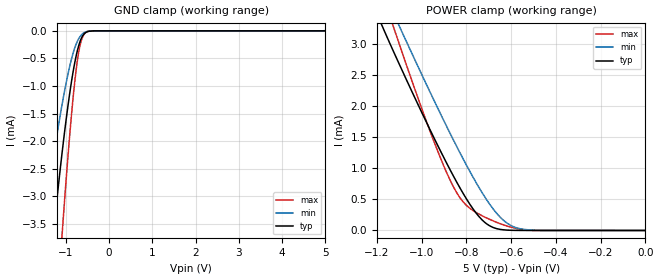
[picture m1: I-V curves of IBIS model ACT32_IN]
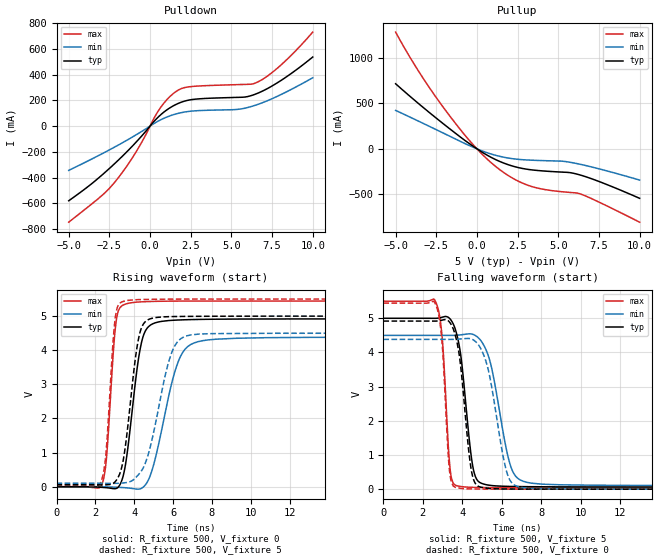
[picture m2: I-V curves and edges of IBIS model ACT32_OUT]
| TEXAS INSTRUMENTS INCORPORATED
| Standard Linear and Logic Group
| IBIS Model of SN74ACT32
| QUADRUPLE 2-INPUT POSITIVE-OR GATES
| This file contains package information for the following:
|  SOIC 14-pin (D) package as [Component] ACT32_D
|  SSOP 14-pin (DB) package as [Component] ACT32_DB
|  PDIP 14-pin (N) package as [Component] ACT32_N
|  TSSOP 14-pin (PW) package as [Component] ACT32_PW
| This device can be powered at the following Vccs:
|  5 volt Vcc
| This file provides unique models under the [Model Selector] for each Vcc.
| For operation at a specific Vcc, select the appropriate model after each
| [Model Selector] keyword.
[IBIS Ver]   3.2
[Comment char]  |_char
[File Name]   sn74act32.ibs
[File Rev]   1.1 | x_die
[Date]   September 5, 2002
[Source]   Data created from TI-SPICE simulations at TI-SLL.
[Notes]   The following is an IBIS list for the ACT32.
   Please contact sllibis@ti.com with questions and
   comments concerning SLL IBIS models.
   This IBIS model is created from a BA (back annotated netlist
[Disclaimer] Property of Texas Instruments Incorporated.  Unauthorized
   reproduction and/or distribution is strictly prohibited.
   This product is protected under copyright law.
   Created  2002, (C) Copyright  2002, Texas Instruments
   Incorporated, All Rights Reserved
   UNLESS THERE IS A SIGNED, WRITTEN AGREEMENT TO THE
   CONTRARY, TEXAS INSTRUMENTS (TI) IS PROVIDING THE IBIS
   MODELS  AND WITHOUT ANY WARRANTY, EXPRESSED OR
   IMPLIED.  TI assumes no liability for:
   1) the accuracy of the IBIS models provided to your
   company;
   2) the proper functioning of these IBIS Models in your
   design or for any resulting applications; or
   3) infringement of patents, copyrights or intellectual
   property rights resulting from your use of these IBIS
   models.
   TI provides IBIS Models as a service to our customers.
   You and your company shall not distribute, sell or give
   these models to anyone else without prior written
   permission from TI.
   TI reserves the right to make changes to our products or
   to discontinue any semiconductor product or service
   without notice, and advises our customers to obtain the
   latest version of relevant information to verify, before
   placing orders, that the information being relied on is
   current.
   Please be aware that your receipt and use of the IBIS
   information provided shall serve as acceptance of these
   terms and conditions.  If you do not accept these terms,
   you should return or destroy the IBIS models and any
   other accompanying information immediately.
| Component ACT32_D 14-pin SOIC
[Component]   ACT32_D
[Manufacturer]   Texas Instruments, Inc.
[Package]
|   typ   min   max
R_pkg   3.100e-02   2.800e-02   3.400e-02
L_pkg   3.109e-09   2.462e-09   3.889e-09
C_pkg   4.730e-13   3.630e-13   6.280e-13
[Pin]   signal_name   model_name   R_pin   L_pin   C_pin
1   1A   ACT32_IN   3.300e-02   3.854e-09   6.220e-13
2   1B   ACT32_IN   3.200e-02   3.188e-09   4.730e-13
3   1Y   ACT32_OUT   2.800e-02   2.462e-09   3.770e-13
4   2A   ACT32_IN   3.100e-02   2.596e-09   3.630e-13
5   2B   ACT32_IN   2.800e-02   2.521e-09   3.720e-13
6   2Y   ACT32_OUT   3.400e-02   3.250e-09   4.760e-13
7   GND   GND   3.400e-02   3.889e-09   6.280e-13
8   3Y   ACT32_OUT   3.400e-02   3.889e-09   6.280e-13
9   3A   ACT32_IN   3.400e-02   3.250e-09   4.760e-13
10   3B   ACT32_IN   2.800e-02   2.521e-09   3.720e-13
11   4Y   ACT32_OUT   3.100e-02   2.596e-09   3.640e-13
12   4A   ACT32_IN   2.800e-02   2.462e-09   3.770e-13
13   4B   ACT32_IN   3.200e-02   3.188e-09   4.730e-13
14   VCC   POWER   3.300e-02   3.854e-09   6.220e-13
| Component ACT32_DB 14-pin SSOP
[Component]   ACT32_DB
[Manufacturer]   Texas Instruments, Inc.
[Package]
|   typ   min   max
R_pkg   4.400e-02   4.100e-02   4.600e-02
L_pkg   3.551e-09   3.258e-09   3.927e-09
C_pkg   4.020e-13   3.600e-13   4.210e-13
[Pin]   signal_name   model_name   R_pin   L_pin   C_pin
1   1A   ACT32_IN   4.600e-02   3.927e-09   4.080e-13
2   1B   ACT32_IN   4.400e-02   3.587e-09   4.210e-13
3   1Y   ACT32_OUT   4.100e-02   3.289e-09   3.980e-13
4   2A   ACT32_IN   4.200e-02   3.258e-09   3.600e-13
5   2B   ACT32_IN   4.100e-02   3.286e-09   4.030e-13
6   2Y   ACT32_OUT   4.400e-02   3.586e-09   4.210e-13
7   GND   GND   4.600e-02   3.927e-09   4.080e-13
8   3Y   ACT32_OUT   4.600e-02   3.927e-09   4.080e-13
9   3A   ACT32_IN   4.400e-02   3.586e-09   4.210e-13
10   3B   ACT32_IN   4.100e-02   3.286e-09   4.030e-13
11   4Y   ACT32_OUT   4.300e-02   3.258e-09   3.600e-13
12   4A   ACT32_IN   4.100e-02   3.289e-09   3.980e-13
13   4B   ACT32_IN   4.400e-02   3.587e-09   4.210e-13
14   VCC   POWER   4.600e-02   3.927e-09   4.080e-13
| Component ACT32_N 14-pin PDIP
[Component]   ACT32_N
[Manufacturer]   Texas Instruments, Inc.
[Package]
|   typ   min   max
R_pkg   4.500e-02   3.700e-02   6.300e-02
L_pkg   5.407e-09   3.922e-09   6.942e-09
C_pkg   3.890e-13   2.050e-13   6.040e-13
[Pin]   signal_name   model_name   R_pin   L_pin   C_pin
1   1A   ACT32_IN   6.300e-02   6.942e-09   6.040e-13
2   1B   ACT32_IN   3.700e-02   6.200e-09   4.060e-13
3   1Y   ACT32_OUT   4.200e-02   4.389e-09   3.220e-13
4   2A   ACT32_IN   3.800e-02   3.922e-09   2.050e-13
5   2B   ACT32_IN   3.900e-02   4.301e-09   2.980e-13
6   2Y   ACT32_OUT   3.800e-02   5.329e-09   3.560e-13
7   GND   GND   5.300e-02   6.510e-09   5.440e-13
8   3Y   ACT32_OUT   5.300e-02   6.437e-09   5.390e-13
9   3A   ACT32_IN   3.900e-02   5.352e-09   3.470e-13
10   3B   ACT32_IN   4.200e-02   4.473e-09   2.970e-13
11   4Y   ACT32_OUT   4.400e-02   4.326e-09   2.250e-13
12   4A   ACT32_IN   4.200e-02   4.295e-09   2.800e-13
13   4B   ACT32_IN   4.200e-02   6.318e-09   4.180e-13
14   VCC   POWER   6.100e-02   6.900e-09   6.030e-13
| Component ACT32_PW 14-pin TSSOP
[Component]   ACT32_PW
[Manufacturer]   Texas Instruments, Inc.
[Package]
|   typ   min   max
R_pkg   3.200e-02   2.900e-02   3.500e-02
L_pkg   2.378e-09   2.170e-09   2.680e-09
C_pkg   3.140e-13   2.700e-13   3.350e-13
[Pin]   signal_name   model_name   R_pin   L_pin   C_pin
1   1A   ACT32_IN   3.300e-02   2.618e-09   3.300e-13
2   1B   ACT32_IN   3.100e-02   2.313e-09   3.170e-13
3   1Y   ACT32_OUT   3.000e-02   2.310e-09   3.140e-13
4   2A   ACT32_IN   3.100e-02   2.173e-09   2.720e-13
5   2B   ACT32_IN   3.000e-02   2.204e-09   3.090e-13
6   2Y   ACT32_OUT   3.200e-02   2.315e-09   3.170e-13
7   GND   GND   3.500e-02   2.680e-09   3.350e-13
8   3Y   ACT32_OUT   3.300e-02   2.640e-09   3.330e-13
9   3A   ACT32_IN   3.400e-02   2.347e-09   3.190e-13
10   3B   ACT32_IN   2.900e-02   2.277e-09   3.130e-13
11   4Y   ACT32_OUT   3.100e-02   2.170e-09   2.700e-13
12   4A   ACT32_IN   3.100e-02   2.244e-09   3.110e-13
13   4B   ACT32_IN   3.300e-02   2.343e-09   3.210e-13
14   VCC   POWER   3.500e-02   2.657e-09   3.320e-13
| Models and submodels in the file (2): ACT32_IN (Input), ACT32_OUT (Output)
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| Model ACT32_IN
| Model ACT32_OUT
[Model]   ACT32_IN
Model_type  Input
Vinl=0.8
Vinh=2.0
| variable   typ   min   max
C_comp   0.80pF   0.70pF   1.25pF
[Temperature Range]   40   100   -40
| Ambient temperature   25   85   -40
[Voltage range]   5   4.5   5.5
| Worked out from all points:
|   GND clamp passes 1 mA (typ) near -0.88 V on its own axis
|   POWER clamp passes 1 mA (typ) near -0.88 V on its own axis
[GND Clamp]
| ACT32_IN
|   Voltage   I(typ)   I(min)   I(max)
-5V       -46.92mA   -30.58mA   -59.62mA
-1.56V    -6.035mA   -3.826mA   -9.528mA
-1.51V    -5.59mA    -3.537mA   -8.882mA
-1.305V   -3.869mA   -2.418mA   -6.312mA
-1.255V   -3.478mA   -2.163mA   -5.708mA
-1.08V    -2.21mA    -1.334mA   -3.692mA
-1.06V    -2.076mA   -1.247mA   -3.474mA
-900mV    -1.111mA   -628.4uA   -1.852mA
-770mV    -508.4uA   -270.1uA   -799.3uA
-670mV    -203.9uA   -108.8uA   -280.1uA
-550mV    -38.99uA   -24.34uA   -40.29uA
5V        16.38nA    4.859uA    150.6nA
[POWER Clamp]
| ACT32_IN
|   Voltage   I(typ)   I(min)   I(max)
-5V       45.74mA    45.24mA    49.64mA
-1.17V    3.235mA    3.838mA    3.746mA
-1.125V   2.87mA     3.482mA    3.262mA
-1.075V   2.477mA    3.09mA     2.732mA
-965mV    1.638mA    2.244mA    1.62mA
-895mV    1.129mA    1.722mA    985.3uA
-840mV    755.6uA    1.327mA    587.5uA
-785mV    423.6uA    951.8uA    357.6uA
-695mV    72.53uA    417uA      176.8uA
-640mV    12.79uA    181.6uA    97.2uA
-585mV    1.851uA    53.91uA    37.94uA
-84.45fV  16.38nA    947.5pA    229.7nA
[Model]   ACT32_OUT
Model_type  Output
Vref =   0
Rref =   500
Cref =   50p
Vmeas =   1.5
| variable   typ   min   max
C_comp   13.36pF   5.61pF   24.96pF
| C_pullup   14.73pF   5.61pF   24.96pF
| C_pulldown   11.98pF   5.98pF   19.94pF
[Temperature Range]   40   100   -40
| Ambient temperature   25   85   -40
[Voltage range]   5   4.5   5.5
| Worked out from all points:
|   slope of the pulldown table from 0 to 0.75 V, typ, clamps not added: 7.64 ohm
|   slope of the pullup table from 0 to 0.75 V, typ, clamps not added: 9.15 ohm
|   rising waveform, R_fixture 500, V_fixture 0: 20-80 % time 637ps typ, 1.06ns min, 373ps max; typ from 0 V to 4.92 V
|   falling waveform, R_fixture 500, V_fixture 5: 20-80 % time 537ps typ, 848ps min, 320ps max; typ from 5 V to 0.063 V
|   rising waveform, R_fixture 500, V_fixture 5: 20-80 % time 612ps typ, 1.02ns min, 364ps max; typ from 0.063 V to 5 V
|   falling waveform, R_fixture 500, V_fixture 0: 20-80 % time 512ps typ, 789ps min, 313ps max; typ from 4.92 V to 0 V
[Pulldown]
| ACT32_OUT
|   Voltage   I(typ)   I(min)   I(max)
-5V       -580.4mA   -344.3mA   -746.8mA
-3V       -385.5mA   -218.2mA   -544mA
-2.135V   -286.7mA   -160.2mA   -430.5mA
-865mV    -125.8mA   -68.55mA   -201.6mA
555mV     76.37mA    42.29mA    127mA
1.47V     159.9mA    89.76mA    256.7mA
1.91V     184.9mA    104mA      290.3mA
2.405V    202.4mA    114.2mA    305.1mA
5.375V    222.9mA    129.7mA    322mA
6.535V    250.9mA    164.4mA    337.7mA
8.04V     353.5mA    244.3mA    473.4mA
10V       536.5mA    375.2mA    730.1mA
[Pullup]
| ACT32_OUT
|   Voltage   I(typ)   I(min)   I(max)
-5V       714.7mA    422.3mA    1.282A
-3.495V   482.8mA    295.7mA    826.6mA
-1.81V    239.1mA    150.5mA    393.9mA
-145mV    17.72mA    11.1mA     28.11mA
570mV     -63.95mA   -39.32mA   -102.7mA
1.285V    -129.4mA   -77.34mA   -212.7mA
2.305V    -195.1mA   -111mA     -333.4mA
3.33V     -230.3mA   -124.6mA   -411.9mA
5.235V    -255.6mA   -135.9mA   -471.4mA
6.175V    -279mA     -163.2mA   -486.7mA
7.215V    -339.4mA   -206.5mA   -560.8mA
10V       -543.6mA   -343.1mA   -805.8mA
[Ramp]
| ACT32_OUT
| variable   typ   min   max
dV/dt_r   2.99/6.47E-10   2.67/1.08E-09   3.29/3.81E-10
dV/dt_f   2.99/5.49E-10   2.66/8.61E-10   3.31/3.31E-10
R_load = 500
[Rising Waveform]
| ACT32_OUT
R_fixture =   500
C_fixture =   0
L_fixture =   0
V_fixture =   0
V_fixture_min = 0
V_fixture_max = 0
|   Time   V(typ)   V(min)   V(max)
0s        1.229nV    2.108nV    825.9pV
2.34ns    -18.49mV   -1.135mV   70.97mV
2.575ns   -28.66mV   -4.756mV   859.9mV
3.08ns    -49.42mV   -15.38mV   4.881V
3.765ns   1.571V     -41.53mV   5.384V
4.235ns   3.804V     -70.16mV   5.414V
4.61ns    4.601V     80.4mV     5.425V
6.285ns   4.887V     3.692V     5.441V
7.545ns   4.905V     4.282V     5.442V
50ns      4.918V     4.383V     5.443V
[Falling Waveform]
| ACT32_OUT
R_fixture =   500
C_fixture =   0
L_fixture =   0
V_fixture =   5
V_fixture_min = 4.5
V_fixture_max = 5.5
|   Time   V(typ)   V(min)   V(max)
0s        5V         4.5V       5.5V
2.685ns   5V         4.5V       5.435V
2.99ns    5.033V     4.5V       4.379V
3.39ns    4.974V     4.499V     552.1mV
3.76ns    4.436V     4.506V     94.67mV
4.56ns    586.6mV    4.524V     52.73mV
5.31ns    120.3mV    3.92V      46.05mV
6.455ns   79.89mV    667.2mV    42.76mV
7.495ns   72.29mV    176.1mV    41.65mV
50ns      63.36mV    104.1mV    40.77mV
[Rising Waveform]
| ACT32_OUT
R_fixture =   500
C_fixture =   0
L_fixture =   0
V_fixture =   5
V_fixture_min = 4.5
V_fixture_max = 5.5
|   Time   V(typ)   V(min)   V(max)
0s        63.36mV    104.1mV    40.77mV
2.305ns   53.43mV    103.2mV    171.7mV
2.55ns    56mV       100.7mV    1.005V
3.03ns    154.2mV    99.47mV    4.972V
3.585ns   1.362V     121.2mV    5.451V
4.085ns   3.865V     272.5mV    5.481V
4.415ns   4.71V      502.1mV    5.488V
5.905ns   4.986V     3.891V     5.498V
6.915ns   4.993V     4.449V     5.499V
50ns      5V         4.5V       5.5V
[Falling Waveform]
| ACT32_OUT
R_fixture =   500
C_fixture =   0
L_fixture =   0
V_fixture =   0
V_fixture_min = 0
V_fixture_max = 0
|   Time   V(typ)   V(min)   V(max)
0s        4.918V     4.383V     5.443V
2.665ns   4.918V     4.383V     5.386V
2.985ns   4.947V     4.382V     4.213V
3.36ns    4.882V     4.382V     502.6mV
3.74ns    4.272V     4.388V     38.96mV
4.47ns    518.5mV    4.391V     7.248mV
5.115ns   38.41mV    3.882V     2.812mV
6.255ns   4.861mV    499.8mV    890.7uV
7.095ns   2.282mV    41.61mV    444.6uV
50ns      -4.631nV   -3.818nV   -6.44nV
